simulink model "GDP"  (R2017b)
settings: Solver=FixedStepDiscrete  StartTime=0.0  StopTime=10.0  FixedStep=0.01  RelTol=1e-3  EnableMultiTasking=on
undefined symbols (not defined in the file): ASWTYPE_FALSE, ASWTYPE_TRUE, CcGDP_DCCANBusOffFltTi_ms, Enum_DCCDCConnSt, Enum_LDPCC2St, GDP_CONST1_NUMB, GDP_RUNTIME_MS
libraries: AIWAYS_Powertrain_BMS_lib x68
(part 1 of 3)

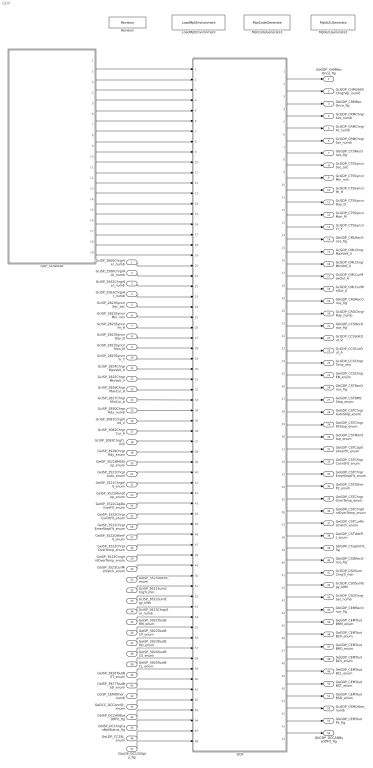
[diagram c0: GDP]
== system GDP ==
  GcISP_2600ChrgrVer_numb : Inport
  GcISP_2560ChrgrAck_numb : Inport  Port=2
  GcISP_2561ChrgrSer_numb : Inport  Port=3
  GcISP_2562ChrgrAr_numb : Inport  Port=4
  GcISP_2823SyncnSec_sec : Inport  Port=5
  GcISP_2823SyncnMin_min : Inport  Port=6
  GcISP_2823SyncnHr_H : Inport  Port=7
  GcISP_2823SyncnDay_D : Inport  Port=8
  GcISP_2823SyncnMon_M : Inport  Port=9
  GcISP_2823SyncnYr_Y : Inport  Port=10
  GcISP_2824ChrgrMaxVolt_V : Inport  Port=11
  GcISP_2825ChrgrMinVolt_V : Inport  Port=12
  GcISP_2826ChrgrMaxCur_A : Inport  Port=13
  GcISP_2827ChrgrMinCur_A : Inport  Port=14
  GcISP_2830ChrgrRdy_numb : Inport  Port=15
  GcISP_3081ChrgrVolt_V : Inport  Port=16
  GcISP_3082ChrgrCur_A : Inport  Port=17
  GcISP_3083ChrgTi_min : Inport  Port=18
  GeISP_3929ChrgrRdy_enum : Inport  Port=19
  GeISP_3521BMSStop_enum : Inport  Port=20
  GeISP_3521ChrgrAuto_enum : Inport  Port=21
  GeISP_3521ChrgrFlt_enum : Inport  Port=22
  GeISP_3521ManStop_enum : Inport  Port=23
  GeISP_3522CapDeliverFlt_enum : Inport  Port=24
  GeISP_3522ChrgrConntFlt_enum : Inport  Port=25
  GeISP_3522ChrgrEmerStopFlt_enum : Inport  Port=26
  GeISP_3522OtherFlt_enum : Inport  Port=27
  GeISP_3522ChrgrOverTemp_enum : Inport  Port=28
  GeISP_3522ChrgrIntOverTemp_enum : Inport  Port=29
  GeISP_3523CurMismatch_enum : Inport  Port=30
  GeISP_3523VoltFlt_enum : Inport  Port=31
  GcISP_3611SumChrgTi_min : Inport  Port=32
  GcISP_3612SumEgy_kWh : Inport  Port=33
  GcISP_3613ChrgrSer_numb : Inport  Port=34
  GeISP_3921ToutBRM_enum : Inport  Port=35
  GeISP_3922ToutBCP_enum : Inport  Port=36
  GeISP_3923ToutBRO_enum : Inport  Port=37
  GeISP_3924ToutBCS_enum : Inport  Port=38
  GeISP_3925ToutBCL_enum : Inport  Port=39
  GeISP_3926ToutBST_enum : Inport  Port=40
  GeISP_3927ToutBSD_enum : Inport  Port=41
  GcISP_CEMOther_numb : Inport  Port=42
  GeDCC_DCConnSt_enum : Inport  Port=43
  GbISP_DCCANBusOffFlt_flg : Inport  Port=44
  GbISP_DCChrgCanNetStatus_flg : Inport  Port=45
  GeLDP_CC2St_enum : Inport  Port=46
  GbLDP_DC12VSply_flg : Inport  Port=47
  DCR : Subsystem
  GDP_Schedule : Stateflow chart  TreatAsAtomicUnit=on
  LoadMptEnvironment : AIWAYS_Powertrain_BMS_lib/Config/LoadMptEnvironment  ProjectName=Comm  SuppierID=NewPlatformUAES
  MptA2LGenerate1 : AIWAYS_Powertrain_BMS_lib/Config/MptA2LGenerate  SystemSampleTime=-1
  MptCodeGenerate1 : AIWAYS_Powertrain_BMS_lib/Config/MptCodeGenerate  SystemSampleTime=-1
  Revision : AIWAYS_Powertrain_BMS_lib/Config/Revision  curVersion='M100C100'  newVersion='M100C100'
  GbGDP_CHMRecOnce_flg : Outport
  GcGDP_CHM2600ChrgrVer_numb : Outport  Port=2
  GbGDP_CRMRecOnce_flg : Outport  Port=3
  GcGDP_CRMChrgrAck_numb : Outport  Port=4
  GcGDP_CRMChrgrAr_numb : Outport  Port=5
  GcGDP_CRMChrgrSer_numb : Outport  Port=6
  GbGDP_CTSRecOnce_flg : Outport  Port=7
  GcGDP_CTSSyncnSec_sec : Outport  Port=8
  GcGDP_CTSSyncnMin_min : Outport  Port=9
  GcGDP_CTSSyncnHr_H : Outport  Port=10
  GcGDP_CTSSyncnDay_D : Outport  Port=11
  GcGDP_CTSSyncnMon_M : Outport  Port=12
  GcGDP_CTSSyncnYr_Y : Outport  Port=13
  GbGDP_CMLRecOnce_flg : Outport  Port=14
  GcGDP_CMLChrgrMaxVolt_V : Outport  Port=15
  GcGDP_CMLChrgrMinVolt_V : Outport  Port=16
  GcGDP_CMLCurMaxOut_A : Outport  Port=17
  GcGDP_CMLCurMinOut_A : Outport  Port=18
  GbGDP_CRORecOnce_flg : Outport  Port=19
  GcGDP_CROChrgrRdy_numb : Outport  Port=20
  GbGDP_CCSRecOnce_flg : Outport  Port=21
  GcGDP_CCSVoltOut_V : Outport  Port=22
  GcGDP_CCSCurOut_A : Outport  Port=23
  GcGDP_CCSChrgrTime_min : Outport  Port=24
  GeGDP_CCSChrgrEN_enum : Outport  Port=25
  GbGDP_CSTRecOnce_flg : Outport  Port=26
  GeGDP_CSTBMSStop_enum : Outport  Port=27
  GeGDP_CSTChrgrAutoStop_enum : Outport  Port=28
  GeGDP_CSTChrgrFltStop_enum : Outport  Port=29
  GeGDP_CSTManStop_enum : Outport  Port=30
  GeGDP_CSTCapDeliverFlt_enum : Outport  Port=31
  GeGDP_CSTChrgrConntFlt_enum : Outport  Port=32
  GeGDP_CSTChrgrEmerStopFlt_enum : Outport  Port=33
  GeGDP_CSTOtherFlt_enum : Outport  Port=34
  GeGDP_CSTChrgrOverTemp_enum : Outport  Port=35
  GeGDP_CSTChrgrIntOverTemp_enum : Outport  Port=36
  GeGDP_CSTCurMismatch_enum : Outport  Port=37
  GeGDP_CSTVoltFlt_enum : Outport  Port=38
  GbGDP_ChrgrInFlt_flg : Outport  Port=39
  GbGDP_CSDRecOnce_flg : Outport  Port=40
  GcGDP_CSDSumChrgTi_min : Outport  Port=41
  GcGDP_CSDSumEgy_kWh : Outport  Port=42
  GcGDP_CSDChrgrSer_numb : Outport  Port=43
  GbGDP_CEMRecOnce_flg : Outport  Port=44
  GeGDP_CEMToutBRM_enum : Outport  Port=45
  GeGDP_CEMToutBCP_enum : Outport  Port=46
  GeGDP_CEMToutBRO_enum : Outport  Port=47
  GeGDP_CEMToutBCS_enum : Outport  Port=48
  GeGDP_CEMToutBCL_enum : Outport  Port=49
  GeGDP_CEMToutBST_enum : Outport  Port=50
  GeGDP_CEMToutBSD_enum : Outport  Port=51
  GcGDP_CEMOther_numb : Outport  Port=52
  GbGDP_CEMToutFlt_flg : Outport  Port=53
  GbGDP_DCCANBusOffFlt_flg : Outport  Port=54
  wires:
  GeISP_3926ToutBST_enum/1 -> DCR/59(GeISP_3926ToutBST_enum)
  GeISP_3921ToutBRM_enum/1 -> DCR/54(GeISP_3921ToutBRM_enum)
  GcISP_2824ChrgrMaxVolt_V/1 -> DCR/30(GcISP_2824ChrgrMaxVolt_V)
  GeISP_3929ChrgrRdy_enum/1 -> DCR/38(GeISP_3929ChrgrRdy_enum)
  GcISP_2827ChrgrMinCur_A/1 -> DCR/33(GcISP_2827ChrgrMinCur_A)
  GcISP_2830ChrgrRdy_numb/1 -> DCR/34(GcISP_2830ChrgrRdy_numb)
  GeISP_3522ChrgrConntFlt_enum/1 -> DCR/44(GeISP_3522ChrgrConntFlt_enum)
  GcISP_3611SumChrgTi_min/1 -> DCR/51(GcISP_3611SumChrgTi_min)
  GcISP_2823SyncnYr_Y/1 -> DCR/29(GcISP_2823SyncnYr_Y)
  GeISP_3521ManStop_enum/1 -> DCR/42(GeISP_3521ManStop_enum)
  GeISP_3522ChrgrIntOverTemp_enum/1 -> DCR/48(GeISP_3522ChrgrIntOverTemp_enum)
  GcISP_3081ChrgrVolt_V/1 -> DCR/35(GcISP_3081ChrgrVolt_V)
  GcISP_2823SyncnHr_H/1 -> DCR/26(GcISP_2823SyncnHr_H)
  GcISP_3613ChrgrSer_numb/1 -> DCR/53(GcISP_3613ChrgrSer_numb)
  GeISP_3522CapDeliverFlt_enum/1 -> DCR/43(GeISP_3522CapDeliverFlt_enum)
  GeISP_3523CurMismatch_enum/1 -> DCR/49(GeISP_3523CurMismatch_enum)
  GeISP_3521BMSStop_enum/1 -> DCR/39(GeISP_3521BMSStop_enum)
  GeISP_3521ChrgrAuto_enum/1 -> DCR/40(GeISP_3521ChrgrAuto_enum)
  GeISP_3925ToutBCL_enum/1 -> DCR/58(GeISP_3925ToutBCL_enum)
  GcISP_2561ChrgrSer_numb/1 -> DCR/22(GcISP_2561ChrgrSer_numb)
  GcISP_2823SyncnMin_min/1 -> DCR/25(GcISP_2823SyncnMin_min)
  GcISP_2823SyncnDay_D/1 -> DCR/27(GcISP_2823SyncnDay_D)
  GcISP_2600ChrgrVer_numb/1 -> DCR/20(GcISP_2600ChrgrVer_numb)
  GcISP_2825ChrgrMinVolt_V/1 -> DCR/31(GcISP_2825ChrgrMinVolt_V)
  GeISP_3923ToutBRO_enum/1 -> DCR/56(GeISP_3923ToutBRO_enum)
  GcISP_2562ChrgrAr_numb/1 -> DCR/23(GcISP_2562ChrgrAr_numb)
  GcISP_2823SyncnSec_sec/1 -> DCR/24(GcISP_2823SyncnSec_sec)
  GcISP_2823SyncnMon_M/1 -> DCR/28(GcISP_2823SyncnMon_M)
  GeISP_3522OtherFlt_enum/1 -> DCR/46(GeISP_3522OtherFlt_enum)
  GcISP_2826ChrgrMaxCur_A/1 -> DCR/32(GcISP_2826ChrgrMaxCur_A)
  GeISP_3521ChrgrFlt_enum/1 -> DCR/41(GeISP_3521ChrgrFlt_enum)
  GeISP_3522ChrgrOverTemp_enum/1 -> DCR/47(GeISP_3522ChrgrOverTemp_enum)
  GeISP_3522ChrgrEmerStopFlt_enum/1 -> DCR/45(GeISP_3522ChrgrEmerStopFlt_enum)
  GcISP_2560ChrgrAck_numb/1 -> DCR/21(GcISP_2560ChrgrAck_numb)
  GcISP_3083ChrgTi_min/1 -> DCR/37(GcISP_3083ChrgTi_min)
  GeISP_3523VoltFlt_enum/1 -> DCR/50(GeISP_3523VoltFlt_enum)
  GcISP_3612SumEgy_kWh/1 -> DCR/52(GcISP_3612SumEgy_kWh)
  GcISP_3082ChrgrCur_A/1 -> DCR/36(GcISP_3082ChrgrCur_A)
  GeISP_3922ToutBCP_enum/1 -> DCR/55(GeISP_3922ToutBCP_enum)
  GeISP_3924ToutBCS_enum/1 -> DCR/57(GeISP_3924ToutBCS_enum)
  GeISP_3927ToutBSD_enum/1 -> DCR/60(GeISP_3927ToutBSD_enum)
  GeDCC_DCConnSt_enum/1 -> DCR/62(GeDCC_DCConnSt_enum)
  GbISP_DCCANBusOffFlt_flg/1 -> DCR/63(GbISP_DCCANBusOffFlt_flg)
  GcISP_CEMOther_numb/1 -> DCR/61(GcISP_CEMOther_numb)
  DCR/14(GbGDP_CMLRecOnce_flg) -> GbGDP_CMLRecOnce_flg/1
  DCR/15(GcGDP_CMLChrgrMaxVolt_V) -> GcGDP_CMLChrgrMaxVolt_V/1
  DCR/16(GcGDP_CMLChrgrMinVolt_V) -> GcGDP_CMLChrgrMinVolt_V/1
  DCR/17(GcGDP_CMLCurMaxOut_A) -> GcGDP_CMLCurMaxOut_A/1
  DCR/18(GcGDP_CMLCurMinOut_A) -> GcGDP_CMLCurMinOut_A/1
  DCR/19(GbGDP_CRORecOnce_flg) -> GbGDP_CRORecOnce_flg/1
  DCR/20(GcGDP_CROChrgrRdy_numb) -> GcGDP_CROChrgrRdy_numb/1
  DCR/21(GbGDP_CCSRecOnce_flg) -> GbGDP_CCSRecOnce_flg/1
  DCR/22(GcGDP_CCSVoltOut_V) -> GcGDP_CCSVoltOut_V/1
  DCR/23(GcGDP_CCSCurOut_A) -> GcGDP_CCSCurOut_A/1
  DCR/24(GcGDP_CCSChrgrTime_min) -> GcGDP_CCSChrgrTime_min/1
  DCR/25(GeGDP_CCSChrgrEN_enum) -> GeGDP_CCSChrgrEN_enum/1
  DCR/26(GbGDP_CSTRecOnce_flg) -> GbGDP_CSTRecOnce_flg/1
  DCR/27(GeGDP_CSTBMSStop_enum) -> GeGDP_CSTBMSStop_enum/1
  DCR/28(GeGDP_CSTChrgrAutoStop_enum) -> GeGDP_CSTChrgrAutoStop_enum/1
  DCR/29(GeGDP_CSTChrgrFltStop_enum) -> GeGDP_CSTChrgrFltStop_enum/1
  DCR/30(GeGDP_CSTManStop_enum) -> GeGDP_CSTManStop_enum/1
  DCR/31(GeGDP_CSTCapDeliverFlt_enum) -> GeGDP_CSTCapDeliverFlt_enum/1
  DCR/32(GeGDP_CSTChrgrConntFlt_enum) -> GeGDP_CSTChrgrConntFlt_enum/1
  DCR/33(GeGDP_CSTChrgrEmerStopFlt_enum) -> GeGDP_CSTChrgrEmerStopFlt_enum/1
  DCR/34(GeGDP_CSTOtherFlt_enum) -> GeGDP_CSTOtherFlt_enum/1
  DCR/35(GeGDP_CSTChrgrOverTemp_enum) -> GeGDP_CSTChrgrOverTemp_enum/1
  DCR/36(GeGDP_CSTChrgrIntOverTemp_enum) -> GeGDP_CSTChrgrIntOverTemp_enum/1
  DCR/37(GeGDP_CSTCurMismatch_enum) -> GeGDP_CSTCurMismatch_enum/1
  DCR/38(GeGDP_CSTVoltFlt_enum) -> GeGDP_CSTVoltFlt_enum/1
  DCR/39(GbGDP_ChrgrInFlt_flg) -> GbGDP_ChrgrInFlt_flg/1
  DCR/40(GbGDP_CSDRecOnce_flg) -> GbGDP_CSDRecOnce_flg/1
  DCR/41(GcGDP_CSDSumChrgTi_min) -> GcGDP_CSDSumChrgTi_min/1
  DCR/42(GcGDP_CSDSumEgy_kWh) -> GcGDP_CSDSumEgy_kWh/1
  DCR/43(GcGDP_CSDChrgrSer_numb) -> GcGDP_CSDChrgrSer_numb/1
  DCR/44(GbGDP_CEMRecOnce_flg) -> GbGDP_CEMRecOnce_flg/1
  DCR/45(GeGDP_CEMToutBRM_enum) -> GeGDP_CEMToutBRM_enum/1
  DCR/46(GeGDP_CEMToutBCP_enum) -> GeGDP_CEMToutBCP_enum/1
  DCR/47(GeGDP_CEMToutBRO_enum) -> GeGDP_CEMToutBRO_enum/1
  DCR/48(GeGDP_CEMToutBCS_enum) -> GeGDP_CEMToutBCS_enum/1
  DCR/49(GeGDP_CEMToutBCL_enum) -> GeGDP_CEMToutBCL_enum/1
  DCR/50(GeGDP_CEMToutBST_enum) -> GeGDP_CEMToutBST_enum/1
  DCR/51(GeGDP_CEMToutBSD_enum) -> GeGDP_CEMToutBSD_enum/1
  DCR/52(GcGDP_CEMOther_numb) -> GcGDP_CEMOther_numb/1
  DCR/53(GbGDP_CEMToutFlt_flg) -> GbGDP_CEMToutFlt_flg/1
  DCR/54(GbGDP_DCCANBusOffFlt_flg) -> GbGDP_DCCANBusOffFlt_flg/1
  DCR/1(GbGDP_CHMRecOnce_flg) -> GbGDP_CHMRecOnce_flg/1
  DCR/2(GcGDP_CHM2600ChrgrVer_numb) -> GcGDP_CHM2600ChrgrVer_numb/1
  DCR/3(GbGDP_CRMRecOnce_flg) -> GbGDP_CRMRecOnce_flg/1
  DCR/4(GcGDP_CRMChrgrAck_numb) -> GcGDP_CRMChrgrAck_numb/1
  DCR/5(GcGDP_CRMChrgrAr_numb) -> GcGDP_CRMChrgrAr_numb/1
  DCR/6(GcGDP_CRMChrgrSer_numb) -> GcGDP_CRMChrgrSer_numb/1
  DCR/7(GbGDP_CTSRecOnce_flg) -> GbGDP_CTSRecOnce_flg/1
  DCR/8(GcGDP_CTSSyncnSec_sec) -> GcGDP_CTSSyncnSec_sec/1
  DCR/9(GcGDP_CTSSyncnMin_min) -> GcGDP_CTSSyncnMin_min/1
  DCR/10(GcGDP_CTSSyncnHr_H) -> GcGDP_CTSSyncnHr_H/1
  DCR/11(GcGDP_CTSSyncnDay_D) -> GcGDP_CTSSyncnDay_D/1
  DCR/12(GcGDP_CTSSyncnMon_M) -> GcGDP_CTSSyncnMon_M/1
  DCR/13(GcGDP_CTSSyncnYr_Y) -> GcGDP_CTSSyncnYr_Y/1
  GbISP_DCChrgCanNetStatus_flg/1 -> DCR/64(GbISP_DCChrgCanNetStatus_flg)
  GeLDP_CC2St_enum/1 -> DCR/65(GeLDP_CC2St_enum)
  GbLDP_DC12VSply_flg/1 -> DCR/66(GbLDP_DC12VSply_flg)
  GDP_Schedule/1(GDP_CHM_250ms()) -> DCR/1(GDP_CHM_250ms)
  GDP_Schedule/2(GDP_CRM_250ms()) -> DCR/2(GDP_CRM_250ms)
  GDP_Schedule/3(GDP_CTS_500ms()) -> DCR/3(GDP_CTS_500ms)
  GDP_Schedule/4(GDP_CML_500ms()) -> DCR/4(GDP_CML_500ms)
  GDP_Schedule/5(GDP_CRO_50ms()) -> DCR/5(GDP_CRO_50ms)
  GDP_Schedule/6(GDP_CCS_50ms()) -> DCR/6(GDP_CCS_50ms)
  GDP_Schedule/8(GDP_CSD_250ms()) -> DCR/8(GDP_CSD_250ms)
  GDP_Schedule/9(GDP_CEM_250ms()) -> DCR/9(GDP_CEM_250ms)
  GDP_Schedule/10(GDP_BusOff_10ms()) -> DCR/10(GDP_BusOff_10ms)
  GDP_Schedule/11(GDP_CCSUpdateClr_50ms()) -> DCR/11(GDP_CCSUpdateClr_50ms)
  GDP_Schedule/12(GDP_CEMUpdateClr_250ms()) -> DCR/12(GDP_CEMUpdateClr_250ms)
  GDP_Schedule/13(GDP_CHMUpdateClr_250ms()) -> DCR/13(GDP_CHMUpdateClr_250ms)
  GDP_Schedule/14(GDP_CMLUpdateClr_500ms()) -> DCR/14(GDP_CMLUpdateClr_500ms)
  GDP_Schedule/16(GDP_CROUpdateClr_50ms()) -> DCR/16(GDP_CROUpdateClr_50ms)
  GDP_Schedule/15(GDP_CRMUpdateClr_250ms()) -> DCR/15(GDP_CRMUpdateClr_250ms)
  GDP_Schedule/17(GDP_CSDUpdateClr_250ms()) -> DCR/17(GDP_CSDUpdateClr_250ms)
  GDP_Schedule/18(GDP_CSTUpdateClr_10ms()) -> DCR/18(GDP_CSTUpdateClr_10ms)
  GDP_Schedule/19(GDP_CTSUpdateClr_500ms()) -> DCR/19(GDP_CTSUpdateClr_500ms)
  GDP_Schedule/7(GDP_CST_10ms()) -> DCR/7(GDP_CST_10ms)

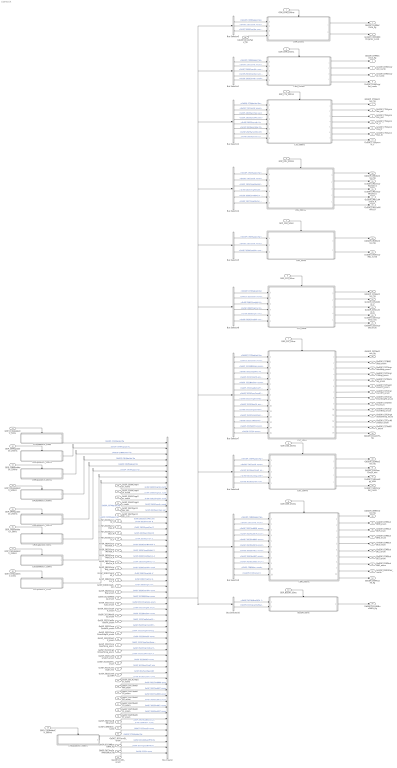
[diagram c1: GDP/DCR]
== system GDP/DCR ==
  GDP_CHM_250ms : Inport
  GDP_CRM_250ms : Inport  Port=2
  GDP_CTS_500ms : Inport  Port=3
  GDP_CML_500ms : Inport  Port=4
  GDP_CRO_50ms : Inport  Port=5
  GDP_CCS_50ms : Inport  Port=6
  GDP_CST_10ms : Inport  Port=7
  GDP_CSD_250ms : Inport  Port=8
  GDP_CEM_250ms : Inport  Port=9
  GDP_BusOff_10ms : Inport  Port=10
  GDP_CCSUpdateClr_50ms : Inport  Port=11
  GDP_CEMUpdateClr_250ms : Inport  Port=12
  GDP_CHMUpdateClr_250ms : Inport  Port=13
  GDP_CMLUpdateClr_500ms : Inport  Port=14
  GDP_CRMUpdateClr_250ms : Inport  Port=15
  GDP_CROUpdateClr_50ms : Inport  Port=16
  GDP_CSDUpdateClr_250ms : Inport  Port=17
  GDP_CSTUpdateClr_10ms : Inport  Port=18
  GDP_CTSUpdateClr_500ms : Inport  Port=19
  GcISP_2600ChrgrVer_numb : Inport  Port=20
  GcISP_2560ChrgrAck_numb : Inport  Port=21
  GcISP_2561ChrgrSer_numb : Inport  Port=22
  GcISP_2562ChrgrAr_numb : Inport  Port=23
  GcISP_2823SyncnSec_sec : Inport  Port=24
  GcISP_2823SyncnMin_min : Inport  Port=25
  GcISP_2823SyncnHr_H : Inport  Port=26
  GcISP_2823SyncnDay_D : Inport  Port=27
  GcISP_2823SyncnMon_M : Inport  Port=28
  GcISP_2823SyncnYr_Y : Inport  Port=29
  GcISP_2824ChrgrMaxVolt_V : Inport  Port=30
  GcISP_2825ChrgrMinVolt_V : Inport  Port=31
  GcISP_2826ChrgrMaxCur_A : Inport  Port=32
  GcISP_2827ChrgrMinCur_A : Inport  Port=33
  GcISP_2830ChrgrRdy_numb : Inport  Port=34
  GcISP_3081ChrgrVolt_V : Inport  Port=35
  GcISP_3082ChrgrCur_A : Inport  Port=36
  GcISP_3083ChrgTi_min : Inport  Port=37
  GeISP_3929ChrgrRdy_enum : Inport  Port=38
  GeISP_3521BMSStop_enum : Inport  Port=39
  GeISP_3521ChrgrAuto_enum : Inport  Port=40
  GeISP_3521ChrgrFlt_enum : Inport  Port=41
  GeISP_3521ManStop_enum : Inport  Port=42
  GeISP_3522CapDeliverFlt_enum : Inport  Port=43
  GeISP_3522ChrgrConntFlt_enum : Inport  Port=44
  GeISP_3522ChrgrEmerStopFlt_enum : Inport  Port=45
  GeISP_3522OtherFlt_enum : Inport  Port=46
  GeISP_3522ChrgrOverTemp_enum : Inport  Port=47
  GeISP_3522ChrgrIntOverTemp_enum : Inport  Port=48
  GeISP_3523CurMismatch_enum : Inport  Port=49
  GeISP_3523VoltFlt_enum : Inport  Port=50
  GcISP_3611SumChrgTi_min : Inport  Port=51
  GcISP_3612SumEgy_kWh : Inport  Port=52
  GcISP_3613ChrgrSer_numb : Inport  Port=53
  GeISP_3921ToutBRM_enum : Inport  Port=54
  GeISP_3922ToutBCP_enum : Inport  Port=55
  GeISP_3923ToutBRO_enum : Inport  Port=56
  GeISP_3924ToutBCS_enum : Inport  Port=57
  GeISP_3925ToutBCL_enum : Inport  Port=58
  GeISP_3926ToutBST_enum : Inport  Port=59
  GeISP_3927ToutBSD_enum : Inport  Port=60
  GcISP_CEMOther_numb : Inport  Port=61
  GeDCC_DCConnSt_enum : Inport  Port=62
  GbISP_DCCANBusOffFlt_flg : Inport  Port=63
  GbISP_DCChrgCanNetStatus_flg : Inport  Port=64
  GeLDP_CC2St_enum : Inport  Port=65
  GbLDP_DC12VSply_flg : Inport  Port=66
  Bus Creator : BusCreator  Inputs=55
  Bus Selector1 : BusSelector  OutputSignals=GbGDP_CRMMsgUpd_flg,GeDCC_DCConnSt_enum,GcISP_2560ChrgrAck_numb,GcISP_2561ChrgrSer_numb,GcISP_2562ChrgrAr_numb
  Bus Selector10 : BusSelector  OutputSignals=GbISP_DCCANBusOffFlt_flg,GbISP_DCChrgCanNetStatus_flg
  Bus Selector2 : BusSelector  OutputSignals=GbGDP_CTSMsgUpd_flg,GeDCC_DCConnSt_enum,GcISP_2823SyncnSec_sec,GcISP_2823SyncnMin_min,GcISP_2823SyncnHr_H,GcISP_2823SyncnDay_D,GcISP_2823SyncnMon_M,GcISP_2823SyncnYr_Y
  Bus Selector3 : BusSelector  OutputSignals=GbGDP_CHMMsgUpd_flg,GeDCC_DCConnSt_enum,GcISP_2600ChrgrVer_numb
  Bus Selector4 : BusSelector  OutputSignals=GbGDP_CMLMsgUpd_flg,GeDCC_DCConnSt_enum,GcISP_2824ChrgrMaxVolt_V,GcISP_2825ChrgrMinVolt_V,GcISP_2826ChrgrMaxCur_A,GcISP_2827ChrgrMinCur_A
  Bus Selector5 : BusSelector  OutputSignals=GbGDP_CROMsgUpd_flg,GeDCC_DCConnSt_enum,GcISP_2830ChrgrRdy_numb
  Bus Selector6 : BusSelector  OutputSignals=GbGDP_CCSMsgUpd_flg,GeDCC_DCConnSt_enum,GcISP_3081ChrgrVolt_V,GcISP_3082ChrgrCur_A,GcISP_3083ChrgTi_min,GeISP_3929ChrgrRdy_enum
  Bus Selector7 : BusSelector  OutputSignals=GbGDP_CSTMsgUpd_flg,GeDCC_DCConnSt_enum,GeISP_3521BMSStop_enum,GeISP_3521ChrgrAuto_enum,GeISP_3521ChrgrFlt_enum,GeISP_3521ManStop_enum,GeISP_3522CapDeliverFlt_enum,GeISP_3522ChrgrConntFlt_enum,GeISP_3522ChrgrEmerStopFlt_enum,GeISP_3522OtherFlt_enum,GeISP_3522ChrgrOverTemp_enum,GeISP_3522ChrgrIntOverTemp_enum,GeISP_3523CurMismatch_enum,GeISP_3523VoltFlt_enum,GeLDP_CC2St_enum
  Bus Selector8 : BusSelector  OutputSignals=GbGDP_CSDMsgUpd_flg,GeDCC_DCConnSt_enum,GcISP_3611SumChrgTi_min,GcISP_3612SumEgy_kWh,GcISP_3613ChrgrSer_numb
  Bus Selector9 : BusSelector  OutputSignals=GbGDP_CEMMsgUpd_flg,GeDCC_DCConnSt_enum,GeISP_3921ToutBRM_enum,GeISP_3922ToutBCP_enum,GeISP_3923ToutBRO_enum,GeISP_3924ToutBCS_enum,GeISP_3925ToutBCL_enum,GeISP_3926ToutBST_enum,GeISP_3927ToutBSD_enum,GcISP_CEMOther_numb,GeLDP_CC2St_enum
  BusOff_10ms : Subsystem
  CCSUpdateClr_50ms : Subsystem
  CCS_50ms : Subsystem
  CEMUpdateClr_250ms : Subsystem
  CEM_250ms : Subsystem
  CHMUpdateClr_250ms : Subsystem
  CHM_250ms : Subsystem
  CMLUpdateClr_500ms : Subsystem
  CML_500ms : Subsystem
  CRMUpdateClr_250ms : Subsystem
  CRM_250ms : Subsystem
  CROUpdateClr_50ms : Subsystem
  CRO_50ms : Subsystem
  CSDUpdateClr_250ms : Subsystem
  CSD_250ms : Subsystem
  CSTUpdateClr_10ms : Subsystem
  CST_10ms : Subsystem
  CTSUpdateClr_500ms : Subsystem
  CTS_500ms : Subsystem
  GbGDP_CHMRecOnce_flg : Outport
  GcGDP_CHM2600ChrgrVer_numb : Outport  Port=2
  GbGDP_CRMRecOnce_flg : Outport  Port=3
  GcGDP_CRMChrgrAck_numb : Outport  Port=4
  GcGDP_CRMChrgrAr_numb : Outport  Port=5
  GcGDP_CRMChrgrSer_numb : Outport  Port=6
  GbGDP_CTSRecOnce_flg : Outport  Port=7
  GcGDP_CTSSyncnSec_sec : Outport  Port=8
  GcGDP_CTSSyncnMin_min : Outport  Port=9
  GcGDP_CTSSyncnHr_H : Outport  Port=10
  GcGDP_CTSSyncnDay_D : Outport  Port=11
  GcGDP_CTSSyncnMon_M : Outport  Port=12
  GcGDP_CTSSyncnYr_Y : Outport  Port=13
  GbGDP_CMLRecOnce_flg : Outport  Port=14
  GcGDP_CMLChrgrMaxVolt_V : Outport  Port=15
  GcGDP_CMLChrgrMinVolt_V : Outport  Port=16
  GcGDP_CMLCurMaxOut_A : Outport  Port=17
  GcGDP_CMLCurMinOut_A : Outport  Port=18
  GbGDP_CRORecOnce_flg : Outport  Port=19
  GcGDP_CROChrgrRdy_numb : Outport  Port=20
  GbGDP_CCSRecOnce_flg : Outport  Port=21
  GcGDP_CCSVoltOut_V : Outport  Port=22
  GcGDP_CCSCurOut_A : Outport  Port=23
  GcGDP_CCSChrgrTime_min : Outport  Port=24
  GeGDP_CCSChrgrEN_enum : Outport  Port=25
  GbGDP_CSTRecOnce_flg : Outport  Port=26
  GeGDP_CSTBMSStop_enum : Outport  Port=27
  GeGDP_CSTChrgrAutoStop_enum : Outport  Port=28
  GeGDP_CSTChrgrFltStop_enum : Outport  Port=29
  GeGDP_CSTManStop_enum : Outport  Port=30
  GeGDP_CSTCapDeliverFlt_enum : Outport  Port=31
  GeGDP_CSTChrgrConntFlt_enum : Outport  Port=32
  GeGDP_CSTChrgrEmerStopFlt_enum : Outport  Port=33
  GeGDP_CSTOtherFlt_enum : Outport  Port=34
  GeGDP_CSTChrgrOverTemp_enum : Outport  Port=35
  GeGDP_CSTChrgrIntOverTemp_enum : Outport  Port=36
  GeGDP_CSTCurMismatch_enum : Outport  Port=37
  GeGDP_CSTVoltFlt_enum : Outport  Port=38
  GbGDP_ChrgrInFlt_flg : Outport  Port=39
  GbGDP_CSDRecOnce_flg : Outport  Port=40
  GcGDP_CSDSumChrgTi_min : Outport  Port=41
  GcGDP_CSDSumEgy_kWh : Outport  Port=42
  GcGDP_CSDChrgrSer_numb : Outport  Port=43
  GbGDP_CEMRecOnce_flg : Outport  Port=44
  GeGDP_CEMToutBRM_enum : Outport  Port=45
  GeGDP_CEMToutBCP_enum : Outport  Port=46
  GeGDP_CEMToutBRO_enum : Outport  Port=47
  GeGDP_CEMToutBCS_enum : Outport  Port=48
  GeGDP_CEMToutBCL_enum : Outport  Port=49
  GeGDP_CEMToutBST_enum : Outport  Port=50
  GeGDP_CEMToutBSD_enum : Outport  Port=51
  GcGDP_CEMOther_numb : Outport  Port=52
  GbGDP_CEMToutFlt_flg : Outport  Port=53
  GbGDP_DCCANBusOffFlt_flg : Outport  Port=54
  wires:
  GcISP_2823SyncnMin_min/1 -> Bus Creator/14  "GcISP_2823SyncnMin_min"
  Bus Selector9/6 -> CEM_250ms/6(GeISP_3924ToutBCS_enum)  "<GeISP_3924ToutBCS_enum>"
  CST_10ms/3(GeGDP_CSTChrgrAutoStop_enum) -> GeGDP_CSTChrgrAutoStop_enum/1
  CEM_250ms/4(GeGDP_CEMToutBRO_enum) -> GeGDP_CEMToutBRO_enum/1
  GeISP_3521ChrgrAuto_enum/1 -> Bus Creator/29  "GeISP_3521ChrgrAuto_enum"
  Bus Selector7/13 -> CST_10ms/13(GeISP_3523CurMismatch_enum)  "<GeISP_3523CurMismatch_enum>"
  Bus Selector9/4 -> CEM_250ms/4(GeISP_3922ToutBCP_enum)  "<GeISP_3922ToutBCP_enum>"
  Bus Selector9/1 -> CEM_250ms/1(GbGDP_CEMMsgUpd_flg)  "<GbGDP_CEMMsgUpd_flg>"
  Bus Selector6/5 -> CCS_50ms/5(GcISP_3083ChrgTi_min)  "<GcISP_3083ChrgTi_min>"
  Bus Selector7/9 -> CST_10ms/9(GeISP_3522ChrgrEmerStopFlt_enum)  "<GeISP_3522ChrgrEmerStopFlt_enum>"
  Bus Selector7/6 -> CST_10ms/6(GeISP_3521ManStop_enum)  "<GeISP_3521ManStop_enum>"
  GDP_CML_500ms/1 -> CML_500ms/Trigger
  CEM_250ms/9(GcGDP_CEMOther_numb) -> GcGDP_CEMOther_numb/1
  Bus Selector1/3 -> CRM_250ms/3(GcISP_2560ChrgrAck_numb)  "<GcISP_2560ChrgrAck_numb>"
  CML_500ms/4(GcGDP_CMLCurMaxOut_A) -> GcGDP_CMLCurMaxOut_A/1
  GeISP_3523VoltFlt_enum/1 -> Bus Creator/39  "GeISP_3523VoltFlt_enum"
  GcISP_3082ChrgrCur_A/1 -> Bus Creator/25  "GcISP_3082ChrgrCur_A"
  Bus Selector9/9 -> CEM_250ms/9(GeISP_3927ToutBSD_enum)  "<GeISP_3927ToutBSD_enum>"
  GcISP_2560ChrgrAck_numb/1 -> Bus Creator/10  "GcISP_2560ChrgrAck_numb"
  CSD_250ms/2(GcGDP_CSDSumChrgTi_min) -> GcGDP_CSDSumChrgTi_min/1
  GeISP_3521BMSStop_enum/1 -> Bus Creator/28  "GeISP_3521BMSStop_enum"
  Bus Selector2/3 -> CTS_500ms/3(GcISP_2823SyncnSec_sec)  "<GcISP_2823SyncnSec_sec>"
  GeISP_3927ToutBSD_enum/1 -> Bus Creator/49  "GeISP_3927ToutBSD_enum"
  GcISP_2827ChrgrMinCur_A/1 -> Bus Creator/22  "GcISP_2827ChrgrMinCur_A"
  CEM_250ms/6(GeGDP_CEMToutBCL_enum) -> GeGDP_CEMToutBCL_enum/1
  CRO_50ms/1(GbGDP_CRORecOnce_flg) -> GbGDP_CRORecOnce_flg/1
  GDP_CEM_250ms/1 -> CEM_250ms/Trigger
  CMLUpdateClr_500ms/1(GbGDP_CMLMsgUpd_flg) -> Bus Creator/4  "GbGDP_CMLMsgUpd_flg"
  Bus Selector3/2 -> CHM_250ms/2(GeDCC_DCConnSt_enum)  "<GeDCC_DCConnSt_enum>"
  CCS_50ms/2(GcGDP_CCSVoltOut_V) -> GcGDP_CCSVoltOut_V/1
  CSD_250ms/4(GcGDP_CSDChrgrSer_numb) -> GcGDP_CSDChrgrSer_numb/1
  Bus Selector4/4 -> CML_500ms/4(GcISP_2825ChrgrMinVolt_V)  "<GcISP_2825ChrgrMinVolt_V>"
  CRMUpdateClr_250ms/1(GbGDP_CRMMsgUpd_flg) -> Bus Creator/5  "GbGDP_CRMMsgUpd_flg"
  Bus Selector7/4 -> CST_10ms/4(GeISP_3521ChrgrAuto_enum)  "<GeISP_3521ChrgrAuto_enum>"
  CST_10ms/12(GeGDP_CSTCurMismatch_enum) -> GeGDP_CSTCurMismatch_enum/1
  Bus Creator/1 -> Bus Selector3/1, Bus Selector1/1, Bus Selector2/1, Bus Selector4/1, Bus Selector5/1, Bus Selector6/1, Bus Selector7/1, Bus Selector8/1, Bus Selector9/1, Bus Selector10/1
  GeISP_3522ChrgrEmerStopFlt_enum/1 -> Bus Creator/34  "GeISP_3522ChrgrEmerStopFlt_enum"
  CML_500ms/5(GcGDP_CMLCurMinOut_A) -> GcGDP_CMLCurMinOut_A/1
  Bus Selector2/1 -> CTS_500ms/1(GbGDP_CTSMsgUpd_flg)  "<GbGDP_CTSMsgUpd_flg>"
  Bus Selector4/3 -> CML_500ms/3(GcISP_2824ChrgrMaxVolt_V)  "<GcISP_2824ChrgrMaxVolt_V>"
  CST_10ms/2(GeGDP_CSTBMSStop_enum) -> GeGDP_CSTBMSStop_enum/1
  CHMUpdateClr_250ms/1(GbGDP_CHMMsgUpd_flg) -> Bus Creator/3  "GbGDP_CHMMsgUpd_flg"
  GcISP_3612SumEgy_kWh/1 -> Bus Creator/41  "GcISP_3612SumEgy_kWh"
  Bus Selector7/5 -> CST_10ms/5(GeISP_3521ChrgrFlt_enum)  "<GeISP_3521ChrgrFlt_enum>"
  CST_10ms/6(GeGDP_CSTCapDeliverFlt_enum) -> GeGDP_CSTCapDeliverFlt_enum/1
  CST_10ms/5(GeGDP_CSTManStop_enum) -> GeGDP_CSTManStop_enum/1
  Bus Selector6/4 -> CCS_50ms/4(GcISP_3082ChrgrCur_A)  "<GcISP_3082ChrgrCur_A>"
  Bus Selector7/7 -> CST_10ms/7(GeISP_3522CapDeliverFlt_enum)  "<GeISP_3522CapDeliverFlt_enum>"
  CEM_250ms/2(GeGDP_CEMToutBRM_enum) -> GeGDP_CEMToutBRM_enum/1
  CML_500ms/1(GbGDP_CMLRecOnce_flg) -> GbGDP_CMLRecOnce_flg/1
  CST_10ms/8(GeGDP_CSTChrgrEmerStopFlt_enum) -> GeGDP_CSTChrgrEmerStopFlt_enum/1
  CST_10ms/9(GeGDP_CSTOtherFlt_enum) -> GeGDP_CSTOtherFlt_enum/1
  Bus Selector6/6 -> CCS_50ms/6(GeISP_3929ChrgrRdy_enum)  "<GeISP_3929ChrgrRdy_enum>"
  GcISP_2823SyncnHr_H/1 -> Bus Creator/15  "GcISP_2823SyncnHr_H"
  GDP_CRO_50ms/1 -> CRO_50ms/Trigger
  GDP_CTS_500ms/1 -> CTS_500ms/Trigger
  GeISP_3522ChrgrIntOverTemp_enum/1 -> Bus Creator/37  "GeISP_3522ChrgrIntOverTemp_enum"
  CRM_250ms/4(GcGDP_CRMChrgrSer_numb) -> GcGDP_CRMChrgrSer_numb/1
  CSD_250ms/3(GcGDP_CSDSumEgy_kWh) -> GcGDP_CSDSumEgy_kWh/1
  CTS_500ms/1(GbGDP_CTSRecOnce_flg) -> GbGDP_CTSRecOnce_flg/1
  CML_500ms/2(GcGDP_CMLChrgrMaxVolt_V) -> GcGDP_CMLChrgrMaxVolt_V/1
  Bus Selector7/12 -> CST_10ms/12(GeISP_3522ChrgrIntOverTemp_enum)  "<GeISP_3522ChrgrIntOverTemp_enum>"
  Bus Selector1/1 -> CRM_250ms/1(GbGDP_CRMMsgUpd_flg)  "<GbGDP_CRMMsgUpd_flg>"
  Bus Selector7/14 -> CST_10ms/14(GeISP_3523VoltFlt_enum)  "<GeISP_3523VoltFlt_enum>"
  CTS_500ms/6(GcGDP_CTSSyncnMon_M) -> GcGDP_CTSSyncnMon_M/1
  Bus Selector7/1 -> CST_10ms/1(GbGDP_CSTMsgUpd_flg)  "<GbGDP_CSTMsgUpd_flg>"
  GcISP_2826ChrgrMaxCur_A/1 -> Bus Creator/21  "GcISP_2826ChrgrMaxCur_A"
  GcISP_2825ChrgrMinVolt_V/1 -> Bus Creator/20  "GcISP_2825ChrgrMinVolt_V"
  CST_10ms/7(GeGDP_CSTChrgrConntFlt_enum) -> GeGDP_CSTChrgrConntFlt_enum/1
  GeISP_3522OtherFlt_enum/1 -> Bus Creator/35  "GeISP_3522OtherFlt_enum"
  GeISP_3922ToutBCP_enum/1 -> Bus Creator/44  "GeISP_3922ToutBCP_enum"
  GeISP_3929ChrgrRdy_enum/1 -> Bus Creator/27  "GeISP_3929ChrgrRdy_enum"
  CST_10ms/4(GeGDP_CSTChrgrFltStop_enum) -> GeGDP_CSTChrgrFltStop_enum/1
  GcISP_3613ChrgrSer_numb/1 -> Bus Creator/42  "GcISP_3613ChrgrSer_numb"
  GDP_CRM_250ms/1 -> CRM_250ms/Trigger
  GeISP_3926ToutBST_enum/1 -> Bus Creator/48  "GeISP_3926ToutBST_enum"
  CST_10ms/13(GeGDP_CSTVoltFlt_enum) -> GeGDP_CSTVoltFlt_enum/1
  Bus Selector8/2 -> CSD_250ms/2(GeDCC_DCConnSt_enum)  "<GeDCC_DCConnSt_enum>"
  Bus Selector6/1 -> CCS_50ms/1(GbGDP_CCSMsgUpd_flg)  "<GbGDP_CCSMsgUpd_flg>"
  CEM_250ms/5(GeGDP_CEMToutBCS_enum) -> GeGDP_CEMToutBCS_enum/1
  Bus Selector9/2 -> CEM_250ms/2(GeDCC_DCConnSt_enum)  "<GeDCC_DCConnSt_enum>"
  CCS_50ms/5(GeGDP_CCSChrgrEN_enum) -> GeGDP_CCSChrgrEN_enum/1
  CEM_250ms/7(GeGDP_CEMToutBST_enum) -> GeGDP_CEMToutBST_enum/1
  Bus Selector8/1 -> CSD_250ms/1(GbGDP_CSDMsgUpd_flg)  "<GbGDP_CSDMsgUpd_flg>"
  GcISP_2600ChrgrVer_numb/1 -> Bus Creator/9  "GcISP_2600ChrgrVer_numb"
  Bus Selector6/2 -> CCS_50ms/2(GeDCC_DCConnSt_enum)  "<GeDCC_DCConnSt_enum>"
  GcISP_2823SyncnYr_Y/1 -> Bus Creator/18  "GcISP_2823SyncnYr_Y"
  CTS_500ms/5(GcGDP_CTSSyncnDay_D) -> GcGDP_CTSSyncnDay_D/1
  GDP_CEMUpdateClr_250ms/1 -> CEMUpdateClr_250ms/Trigger
  GeISP_3522ChrgrOverTemp_enum/1 -> Bus Creator/36  "GeISP_3522ChrgrOverTemp_enum"
  Bus Selector7/11 -> CST_10ms/11(GeISP_3522ChrgrOverTemp_enum)  "<GeISP_3522ChrgrOverTemp_enum>"
  Bus Selector1/4 -> CRM_250ms/4(GcISP_2561ChrgrSer_numb)  "<GcISP_2561ChrgrSer_numb>"
  Bus Selector8/4 -> CSD_250ms/4(GcISP_3612SumEgy_kWh)  "<GcISP_3612SumEgy_kWh>"
  CSD_250ms/1(GbGDP_CSDRecOnce_flg) -> GbGDP_CSDRecOnce_flg/1
  CSTUpdateClr_10ms/1(GbGDP_CSTMsgUpd_flg) -> Bus Creator/8  "GbGDP_CSTMsgUpd_flg"
  CEM_250ms/1(GbGDP_CEMRecOnce_flg) -> GbGDP_CEMRecOnce_flg/1
  Bus Selector4/2 -> CML_500ms/2(GeDCC_DCConnSt_enum)  "<GeDCC_DCConnSt_enum>"
  CST_10ms/11(GeGDP_CSTChrgrIntOverTemp_enum) -> GeGDP_CSTChrgrIntOverTemp_enum/1
  GcISP_3083ChrgTi_min/1 -> Bus Creator/26  "GcISP_3083ChrgTi_min"
  GcISP_CEMOther_numb/1 -> Bus Creator/50  "GcISP_CEMOther_numb"
  GbISP_DCCANBusOffFlt_flg/1 -> Bus Creator/53  "GbISP_DCCANBusOffFlt_flg"
  Bus Selector7/2 -> CST_10ms/2(GeDCC_DCConnSt_enum)  "<GeDCC_DCConnSt_enum>"
  Bus Selector4/5 -> CML_500ms/5(GcISP_2826ChrgrMaxCur_A)  "<GcISP_2826ChrgrMaxCur_A>"
  Bus Selector4/6 -> CML_500ms/6(GcISP_2827ChrgrMinCur_A)  "<GcISP_2827ChrgrMinCur_A>"
  Bus Selector3/3 -> CHM_250ms/3(GcISP_2600ChrgrVer_numb)  "<GcISP_2600ChrgrVer_numb>"
  CEMUpdateClr_250ms/1(GbGDP_CEMMsgUpd_flg) -> Bus Creator/2  "GbGDP_CEMMsgUpd_flg"
  Bus Selector1/2 -> CRM_250ms/2(GeDCC_DCConnSt_enum)  "<GeDCC_DCConnSt_enum>"
  GcISP_2823SyncnSec_sec/1 -> Bus Creator/13  "GcISP_2823SyncnSec_sec"
  Bus Selector4/1 -> CML_500ms/1(GbGDP_CMLMsgUpd_flg)  "<GbGDP_CMLMsgUpd_flg>"
  CHM_250ms/1(GbGDP_CHMRecOnce_flg) -> GbGDP_CHMRecOnce_flg/1
  Bus Selector1/5 -> CRM_250ms/5(GcISP_2562ChrgrAr_numb)  "<GcISP_2562ChrgrAr_numb>"
  Bus Selector6/3 -> CCS_50ms/3(GcISP_3081ChrgrVolt_V)  "<GcISP_3081ChrgrVolt_V>"
  Bus Selector9/7 -> CEM_250ms/7(GeISP_3925ToutBCL_enum)  "<GeISP_3925ToutBCL_enum>"
  GDP_CMLUpdateClr_500ms/1 -> CMLUpdateClr_500ms/Trigger
  CST_10ms/1(GbGDP_CSTRecOnce_flg) -> GbGDP_CSTRecOnce_flg/1
  BusOff_10ms/1(GbGDP_DCCANBusOffFlt_flg) -> GbGDP_DCCANBusOffFlt_flg/1
  GeISP_3925ToutBCL_enum/1 -> Bus Creator/47  "GeISP_3925ToutBCL_enum"
  Bus Selector5/2 -> CRO_50ms/2(GeDCC_DCConnSt_enum)  "<GeDCC_DCConnSt_enum>"
  GcISP_3611SumChrgTi_min/1 -> Bus Creator/40  "GcISP_3611SumChrgTi_min"
  Bus Selector7/8 -> CST_10ms/8(GeISP_3522ChrgrConntFlt_enum)  "<GeISP_3522ChrgrConntFlt_enum>"
  CHM_250ms/2(GcGDP_CHM2600ChrgrVer_numb) -> GcGDP_CHM2600ChrgrVer_numb/1
  GeISP_3923ToutBRO_enum/1 -> Bus Creator/45  "GeISP_3923ToutBRO_enum"
  GcISP_3081ChrgrVolt_V/1 -> Bus Creator/24  "GcISP_3081ChrgrVolt_V"
  CCS_50ms/1(GbGDP_CCSRecOnce_flg) -> GbGDP_CCSRecOnce_flg/1
  CTS_500ms/2(GcGDP_CTSSyncnSec_sec) -> GcGDP_CTSSyncnSec_sec/1
  CRM_250ms/3(GcGDP_CRMChrgrAr_numb) -> GcGDP_CRMChrgrAr_numb/1
  CSDUpdateClr_250ms/1(GbGDP_CSDMsgUpd_flg) -> Bus Creator/7  "GbGDP_CSDMsgUpd_flg"
  Bus Selector2/8 -> CTS_500ms/8(GcISP_2823SyncnYr_Y)  "<GcISP_2823SyncnYr_Y>"
  GDP_CSD_250ms/1 -> CSD_250ms/Trigger
  CRM_250ms/1(GbGDP_CRMRecOnce_flg) -> GbGDP_CRMRecOnce_flg/1
  Bus Selector9/5 -> CEM_250ms/5(GeISP_3923ToutBRO_enum)  "<GeISP_3923ToutBRO_enum>"
  GcISP_2830ChrgrRdy_numb/1 -> Bus Creator/23  "GcISP_2830ChrgrRdy_numb"
  CCS_50ms/4(GcGDP_CCSChrgrTime_min) -> GcGDP_CCSChrgrTime_min/1
  CRM_250ms/2(GcGDP_CRMChrgrAck_numb) -> GcGDP_CRMChrgrAck_numb/1
  Bus Selector5/1 -> CRO_50ms/1(GbGDP_CROMsgUpd_flg)  "<GbGDP_CROMsgUpd_flg>"
  GeISP_3521ManStop_enum/1 -> Bus Creator/31  "GeISP_3521ManStop_enum"
  Bus Selector2/6 -> CTS_500ms/6(GcISP_2823SyncnDay_D)  "<GcISP_2823SyncnDay_D>"
  GeDCC_DCConnSt_enum/1 -> Bus Creator/51  "GeDCC_DCConnSt_enum"
  Bus Selector9/10 -> CEM_250ms/10(GcISP_CEMOther_numb)  "<GcISP_CEMOther_numb>"
  CML_500ms/3(GcGDP_CMLChrgrMinVolt_V) -> GcGDP_CMLChrgrMinVolt_V/1
  Bus Selector10/1 -> BusOff_10ms/1(GbISP_DCCANBusOffFlt_flg)  "<GbISP_DCCANBusOffFlt_flg>"
  CRO_50ms/2(GcGDP_CROChrgrRdy_numb) -> GcGDP_CROChrgrRdy_numb/1
  Bus Selector7/3 -> CST_10ms/3(GeISP_3521BMSStop_enum)  "<GeISP_3521BMSStop_enum>"
  CCSUpdateClr_50ms/1(GbGDP_CCSMsgUpd_flg) -> Bus Creator/1  "GbGDP_CCSMsgUpd_flg"
  CEM_250ms/3(GeGDP_CEMToutBCP_enum) -> GeGDP_CEMToutBCP_enum/1
  CROUpdateClr_50ms/1(GbGDP_CROMsgUpd_flg) -> Bus Creator/6  "GbGDP_CROMsgUpd_flg"
  Bus Selector8/5 -> CSD_250ms/5(GcISP_3613ChrgrSer_numb)  "<GcISP_3613ChrgrSer_numb>"
  Bus Selector5/3 -> CRO_50ms/3(GcISP_2830ChrgrRdy_numb)  "<GcISP_2830ChrgrRdy_numb>"
  Bus Selector3/1 -> CHM_250ms/1(GbGDP_CHMMsgUpd_flg)  "<GbGDP_CHMMsgUpd_flg>"
  GDP_CTSUpdateClr_500ms/1 -> CTSUpdateClr_500ms/Trigger
  Bus Selector9/3 -> CEM_250ms/3(GeISP_3921ToutBRM_enum)  "<GeISP_3921ToutBRM_enum>"
  GDP_CHM_250ms/1 -> CHM_250ms/Trigger
  GcISP_2561ChrgrSer_numb/1 -> Bus Creator/11  "GcISP_2561ChrgrSer_numb"
  Bus Selector2/7 -> CTS_500ms/7(GcISP_2823SyncnMon_M)  "<GcISP_2823SyncnMon_M>"
  CST_10ms/14(GbGDP_ChrgrInFlt_flg) -> GbGDP_ChrgrInFlt_flg/1
  Bus Selector9/8 -> CEM_250ms/8(GeISP_3926ToutBST_enum)  "<GeISP_3926ToutBST_enum>"
  GcISP_2562ChrgrAr_numb/1 -> Bus Creator/12  "GcISP_2562ChrgrAr_numb"
  GDP_CCSUpdateClr_50ms/1 -> CCSUpdateClr_50ms/Trigger
  GcISP_2823SyncnDay_D/1 -> Bus Creator/16  "GcISP_2823SyncnDay_D"
  CTSUpdateClr_500ms/1(GbGDP_CTSMsgUpd_flg) -> Bus Creator/52  "GbGDP_CTSMsgUpd_flg"
  GDP_CSTUpdateClr_10ms/1 -> CSTUpdateClr_10ms/Trigger
  CEM_250ms/10(GbGDP_CEMToutFlt_flg) -> GbGDP_CEMToutFlt_flg/1
  Bus Selector7/10 -> CST_10ms/10(GeISP_3522OtherFlt_enum)  "<GeISP_3522OtherFlt_enum>"
  GDP_CROUpdateClr_50ms/1 -> CROUpdateClr_50ms/Trigger
  GeISP_3924ToutBCS_enum/1 -> Bus Creator/46  "GeISP_3924ToutBCS_enum"
  GDP_CST_10ms/1 -> CST_10ms/Trigger
  CCS_50ms/3(GcGDP_CCSCurOut_A) -> GcGDP_CCSCurOut_A/1
  GDP_CCS_50ms/1 -> CCS_50ms/Trigger
  GDP_CRMUpdateClr_250ms/1 -> CRMUpdateClr_250ms/Trigger
  CTS_500ms/7(GcGDP_CTSSyncnYr_Y) -> GcGDP_CTSSyncnYr_Y/1
  GcISP_2824ChrgrMaxVolt_V/1 -> Bus Creator/19  "GcISP_2824ChrgrMaxVolt_V"
  GcISP_2823SyncnMon_M/1 -> Bus Creator/17  "GcISP_2823SyncnMon_M"
  GeISP_3921ToutBRM_enum/1 -> Bus Creator/43  "GeISP_3921ToutBRM_enum"
  GeISP_3521ChrgrFlt_enum/1 -> Bus Creator/30  "GeISP_3521ChrgrFlt_enum"
  Bus Selector2/4 -> CTS_500ms/4(GcISP_2823SyncnMin_min)  "<GcISP_2823SyncnMin_min>"
  CEM_250ms/8(GeGDP_CEMToutBSD_enum) -> GeGDP_CEMToutBSD_enum/1
  CST_10ms/10(GeGDP_CSTChrgrOverTemp_enum) -> GeGDP_CSTChrgrOverTemp_enum/1
  GDP_CSDUpdateClr_250ms/1 -> CSDUpdateClr_250ms/Trigger
  CTS_500ms/3(GcGDP_CTSSyncnMin_min) -> GcGDP_CTSSyncnMin_min/1
  GDP_CHMUpdateClr_250ms/1 -> CHMUpdateClr_250ms/Trigger
  Bus Selector2/5 -> CTS_500ms/5(GcISP_2823SyncnHr_H)  "<GcISP_2823SyncnHr_H>"
  GeISP_3522ChrgrConntFlt_enum/1 -> Bus Creator/33  "GeISP_3522ChrgrConntFlt_enum"
  GDP_BusOff_10ms/1 -> BusOff_10ms/Trigger
  GeISP_3522CapDeliverFlt_enum/1 -> Bus Creator/32  "GeISP_3522CapDeliverFlt_enum"
  Bus Selector8/3 -> CSD_250ms/3(GcISP_3611SumChrgTi_min)  "<GcISP_3611SumChrgTi_min>"
  CTS_500ms/4(GcGDP_CTSSyncnHr_H) -> GcGDP_CTSSyncnHr_H/1
  GeISP_3523CurMismatch_enum/1 -> Bus Creator/38  "GeISP_3523CurMismatch_enum"
  Bus Selector2/2 -> CTS_500ms/2(GeDCC_DCConnSt_enum)  "<GeDCC_DCConnSt_enum>"
  GbISP_DCChrgCanNetStatus_flg/1 -> Bus Creator/54  "GbISP_DCChrgCanNetStatus_flg"
  Bus Selector10/2 -> BusOff_10ms/2(GbISP_DCChrgCanNetStatus_flg)  "<GbISP_DCChrgCanNetStatus_flg>"
  GeLDP_CC2St_enum/1 -> Bus Creator/55  "GeLDP_CC2St_enum"
  Bus Selector7/15 -> CST_10ms/15(GeLDP_CC2St_enum)  "<GeLDP_CC2St_enum>"
  Bus Selector9/11 -> CEM_250ms/11(GeLDP_CC2St_enum)  "<GeLDP_CC2St_enum>"
  GbLDP_DC12VSply_flg/1 -> CHM_250ms/4(GbLDP_DC12VSply_flg)

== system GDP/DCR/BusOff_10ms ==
  GbISP_DCCANBusOffFlt_flg : Inport
  GbISP_DCChrgCanNetStatus_flg : Inport  Port=2
  GDP_BusOff_10ms : TriggerPort  TriggerType=function-call  VariantControl=(inherit)
  BusOff_10ms_sys : Subsystem
  GbGDP_DCCANBusOffFlt_flg : Outport
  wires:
  BusOff_10ms_sys/1(GbGDP_DCCANBusOffFlt_flg) -> GbGDP_DCCANBusOffFlt_flg/1
  GbISP_DCCANBusOffFlt_flg/1 -> BusOff_10ms_sys/1(GbISP_DCCANBusOffFlt_flg)
  GbISP_DCChrgCanNetStatus_flg/1 -> BusOff_10ms_sys/2(GbISP_DCChrgCanNetStatus_flg)

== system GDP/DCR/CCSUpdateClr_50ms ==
  GDP_CCSUpdateClr_50ms : TriggerPort  TriggerType=function-call  VariantControl=(inherit)
  CCSUpdateClr_50ms_sys : Subsystem
  GbGDP_CCSMsgUpd_flg : Outport
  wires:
  CCSUpdateClr_50ms_sys/1(GbGDP_CCSMsgUpd_flg) -> GbGDP_CCSMsgUpd_flg/1

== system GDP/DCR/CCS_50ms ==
  GbGDP_CCSMsgUpd_flg : Inport
  GeDCC_DCConnSt_enum : Inport  Port=2
  GcISP_3081ChrgrVolt_V : Inport  Port=3
  GcISP_3082ChrgrCur_A : Inport  Port=4
  GcISP_3083ChrgTi_min : Inport  Port=5
  GeISP_3929ChrgrRdy_enum : Inport  Port=6
  GDP_CCS_50ms : TriggerPort  TriggerType=function-call  VariantControl=(inherit)
  CCS_50ms_sys : Subsystem
  GbGDP_CCSRecOnce_flg : Outport
  GcGDP_CCSVoltOut_V : Outport  Port=2
  GcGDP_CCSCurOut_A : Outport  Port=3
  GcGDP_CCSChrgrTime_min : Outport  Port=4
  GeGDP_CCSChrgrEN_enum : Outport  Port=5
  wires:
  GbGDP_CCSMsgUpd_flg/1 -> CCS_50ms_sys/1(GbGDP_CCSMsgUpd_flg)
  GeDCC_DCConnSt_enum/1 -> CCS_50ms_sys/2(GeDCC_DCConnSt_enum)
  GeISP_3929ChrgrRdy_enum/1 -> CCS_50ms_sys/6(GeISP_3929ChrgrRdy_enum)
  GcISP_3081ChrgrVolt_V/1 -> CCS_50ms_sys/3(GcISP_3081ChrgrVolt_V)
  GcISP_3083ChrgTi_min/1 -> CCS_50ms_sys/5(GcISP_3083ChrgTi_min)
  GcISP_3082ChrgrCur_A/1 -> CCS_50ms_sys/4(GcISP_3082ChrgrCur_A)
  CCS_50ms_sys/1(GbGDP_CCSRecOnce_flg) -> GbGDP_CCSRecOnce_flg/1
  CCS_50ms_sys/2(GcGDP_CCSVoltOut_V) -> GcGDP_CCSVoltOut_V/1
  CCS_50ms_sys/3(GcGDP_CCSCurOut_A) -> GcGDP_CCSCurOut_A/1
  CCS_50ms_sys/4(GcGDP_CCSChrgrTime_min) -> GcGDP_CCSChrgrTime_min/1
  CCS_50ms_sys/5(GeGDP_CCSChrgrEN_enum) -> GeGDP_CCSChrgrEN_enum/1

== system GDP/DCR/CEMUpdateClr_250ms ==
  GDP_CEMUpdateClr_250ms : TriggerPort  TriggerType=function-call  VariantControl=(inherit)
  CEMUpdateClr_250ms_sys : Subsystem
  GbGDP_CEMMsgUpd_flg : Outport
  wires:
  CEMUpdateClr_250ms_sys/1(GbGDP_CEMMsgUpd_flg) -> GbGDP_CEMMsgUpd_flg/1

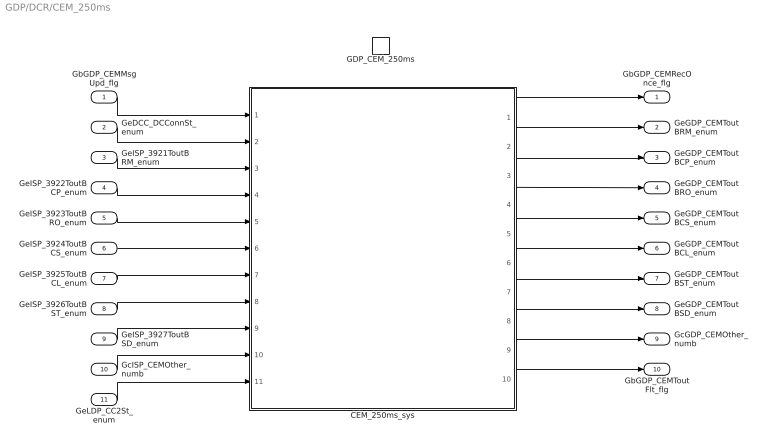
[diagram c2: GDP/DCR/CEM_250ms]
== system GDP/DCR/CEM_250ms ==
  GbGDP_CEMMsgUpd_flg : Inport
  GeDCC_DCConnSt_enum : Inport  Port=2
  GeISP_3921ToutBRM_enum : Inport  Port=3
  GeISP_3922ToutBCP_enum : Inport  Port=4
  GeISP_3923ToutBRO_enum : Inport  Port=5
  GeISP_3924ToutBCS_enum : Inport  Port=6
  GeISP_3925ToutBCL_enum : Inport  Port=7
  GeISP_3926ToutBST_enum : Inport  Port=8
  GeISP_3927ToutBSD_enum : Inport  Port=9
  GcISP_CEMOther_numb : Inport  Port=10
  GeLDP_CC2St_enum : Inport  Port=11
  GDP_CEM_250ms : TriggerPort  TriggerType=function-call  VariantControl=(inherit)
  CEM_250ms_sys : Subsystem
  GbGDP_CEMRecOnce_flg : Outport
  GeGDP_CEMToutBRM_enum : Outport  Port=2
  GeGDP_CEMToutBCP_enum : Outport  Port=3
  GeGDP_CEMToutBRO_enum : Outport  Port=4
  GeGDP_CEMToutBCS_enum : Outport  Port=5
  GeGDP_CEMToutBCL_enum : Outport  Port=6
  GeGDP_CEMToutBST_enum : Outport  Port=7
  GeGDP_CEMToutBSD_enum : Outport  Port=8
  GcGDP_CEMOther_numb : Outport  Port=9
  GbGDP_CEMToutFlt_flg : Outport  Port=10
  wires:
  GbGDP_CEMMsgUpd_flg/1 -> CEM_250ms_sys/1(GbGDP_CEMMsgUpd_flg)
  CEM_250ms_sys/1(GbGDP_CEMRecOnce_flg) -> GbGDP_CEMRecOnce_flg/1
  CEM_250ms_sys/2(GeGDP_CEMToutBRM_enum) -> GeGDP_CEMToutBRM_enum/1
  CEM_250ms_sys/3(GeGDP_CEMToutBCP_enum) -> GeGDP_CEMToutBCP_enum/1
  CEM_250ms_sys/4(GeGDP_CEMToutBRO_enum) -> GeGDP_CEMToutBRO_enum/1
  CEM_250ms_sys/5(GeGDP_CEMToutBCS_enum) -> GeGDP_CEMToutBCS_enum/1
  CEM_250ms_sys/6(GeGDP_CEMToutBCL_enum) -> GeGDP_CEMToutBCL_enum/1
  CEM_250ms_sys/7(GeGDP_CEMToutBST_enum) -> GeGDP_CEMToutBST_enum/1
  CEM_250ms_sys/8(GeGDP_CEMToutBSD_enum) -> GeGDP_CEMToutBSD_enum/1
  CEM_250ms_sys/9(GcGDP_CEMOther_numb) -> GcGDP_CEMOther_numb/1
  GeDCC_DCConnSt_enum/1 -> CEM_250ms_sys/2(GeDCC_DCConnSt_enum)
  GeISP_3924ToutBCS_enum/1 -> CEM_250ms_sys/6(GeISP_3924ToutBCS_enum)
  GeISP_3923ToutBRO_enum/1 -> CEM_250ms_sys/5(GeISP_3923ToutBRO_enum)
  GeISP_3925ToutBCL_enum/1 -> CEM_250ms_sys/7(GeISP_3925ToutBCL_enum)
  GeISP_3922ToutBCP_enum/1 -> CEM_250ms_sys/4(GeISP_3922ToutBCP_enum)
  GeISP_3921ToutBRM_enum/1 -> CEM_250ms_sys/3(GeISP_3921ToutBRM_enum)
  GeISP_3926ToutBST_enum/1 -> CEM_250ms_sys/8(GeISP_3926ToutBST_enum)
  GeISP_3927ToutBSD_enum/1 -> CEM_250ms_sys/9(GeISP_3927ToutBSD_enum)
  GcISP_CEMOther_numb/1 -> CEM_250ms_sys/10(GcISP_CEMOther_numb)
  CEM_250ms_sys/10(GbGDP_CEMToutFlt_flg) -> GbGDP_CEMToutFlt_flg/1
  GeLDP_CC2St_enum/1 -> CEM_250ms_sys/11(GeLDP_CC2St_enum)

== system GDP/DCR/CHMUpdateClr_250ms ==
  GDP_CHMUpdateClr_250ms : TriggerPort  TriggerType=function-call  VariantControl=(inherit)
  CHMUpdateClr_250ms_sys : Subsystem
  GbGDP_CHMMsgUpd_flg : Outport
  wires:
  CHMUpdateClr_250ms_sys/1(GbGDP_CHMMsgUpd_flg) -> GbGDP_CHMMsgUpd_flg/1

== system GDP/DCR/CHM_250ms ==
  GbGDP_CHMMsgUpd_flg : Inport
  GeDCC_DCConnSt_enum : Inport  Port=2
  GcISP_2600ChrgrVer_numb : Inport  Port=3
  GbLDP_DC12VSply_flg : Inport  Port=4
  GDP_CHM_250ms : TriggerPort  TriggerType=function-call  VariantControl=(inherit)
  CHM_250ms_sys : Subsystem
  GbGDP_CHMRecOnce_flg : Outport
  GcGDP_CHM2600ChrgrVer_numb : Outport  Port=2
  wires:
  GbGDP_CHMMsgUpd_flg/1 -> CHM_250ms_sys/1(GbGDP_CHMMsgUpd_flg)
  GeDCC_DCConnSt_enum/1 -> CHM_250ms_sys/2(GeDCC_DCConnSt_enum)
  GcISP_2600ChrgrVer_numb/1 -> CHM_250ms_sys/3(GcISP_2600ChrgrVer_numb)
  CHM_250ms_sys/1(GbGDP_CHMRecOnce_flg) -> GbGDP_CHMRecOnce_flg/1
  CHM_250ms_sys/2(GcGDP_CHM2600ChrgrVer_numb) -> GcGDP_CHM2600ChrgrVer_numb/1
  GbLDP_DC12VSply_flg/1 -> CHM_250ms_sys/4(GbLDP_DC12VSply_flg)

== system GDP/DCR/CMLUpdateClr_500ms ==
  GDP_CMLUpdateClr_500ms : TriggerPort  TriggerType=function-call  VariantControl=(inherit)
  CMLUpdateClr_500ms_sys : Subsystem
  GbGDP_CMLMsgUpd_flg : Outport
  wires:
  CMLUpdateClr_500ms_sys/1(GbGDP_CMLMsgUpd_flg) -> GbGDP_CMLMsgUpd_flg/1

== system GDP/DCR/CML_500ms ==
  GbGDP_CMLMsgUpd_flg : Inport
  GeDCC_DCConnSt_enum : Inport  Port=2
  GcISP_2824ChrgrMaxVolt_V : Inport  Port=3
  GcISP_2825ChrgrMinVolt_V : Inport  Port=4
  GcISP_2826ChrgrMaxCur_A : Inport  Port=5
  GcISP_2827ChrgrMinCur_A : Inport  Port=6
  GDP_CML_500ms : TriggerPort  TriggerType=function-call  VariantControl=(inherit)
  CML_500ms_sys : Subsystem
  GbGDP_CMLRecOnce_flg : Outport
  GcGDP_CMLChrgrMaxVolt_V : Outport  Port=2
  GcGDP_CMLChrgrMinVolt_V : Outport  Port=3
  GcGDP_CMLCurMaxOut_A : Outport  Port=4
  GcGDP_CMLCurMinOut_A : Outport  Port=5
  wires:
  GbGDP_CMLMsgUpd_flg/1 -> CML_500ms_sys/1(GbGDP_CMLMsgUpd_flg)
  GeDCC_DCConnSt_enum/1 -> CML_500ms_sys/2(GeDCC_DCConnSt_enum)
  GcISP_2824ChrgrMaxVolt_V/1 -> CML_500ms_sys/3(GcISP_2824ChrgrMaxVolt_V)
  GcISP_2825ChrgrMinVolt_V/1 -> CML_500ms_sys/4(GcISP_2825ChrgrMinVolt_V)
  GcISP_2826ChrgrMaxCur_A/1 -> CML_500ms_sys/5(GcISP_2826ChrgrMaxCur_A)
  GcISP_2827ChrgrMinCur_A/1 -> CML_500ms_sys/6(GcISP_2827ChrgrMinCur_A)
  CML_500ms_sys/1(GbGDP_CMLRecOnce_flg) -> GbGDP_CMLRecOnce_flg/1
  CML_500ms_sys/2(GcGDP_CMLChrgrMaxVolt_V) -> GcGDP_CMLChrgrMaxVolt_V/1
  CML_500ms_sys/3(GcGDP_CMLChrgrMinVolt_V) -> GcGDP_CMLChrgrMinVolt_V/1
  CML_500ms_sys/4(GcGDP_CMLCurMaxOut_A) -> GcGDP_CMLCurMaxOut_A/1
  CML_500ms_sys/5(GcGDP_CMLCurMinOut_A) -> GcGDP_CMLCurMinOut_A/1

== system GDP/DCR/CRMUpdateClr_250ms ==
  GDP_CRMUpdateClr_250ms : TriggerPort  TriggerType=function-call  VariantControl=(inherit)
  CRMUpdateClr_250ms_sys : Subsystem
  GbGDP_CRMMsgUpd_flg : Outport
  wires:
  CRMUpdateClr_250ms_sys/1(GbGDP_CRMMsgUpd_flg) -> GbGDP_CRMMsgUpd_flg/1

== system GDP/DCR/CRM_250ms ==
  GbGDP_CRMMsgUpd_flg : Inport
  GeDCC_DCConnSt_enum : Inport  Port=2
  GcISP_2560ChrgrAck_numb : Inport  Port=3
  GcISP_2561ChrgrSer_numb : Inport  Port=4
  GcISP_2562ChrgrAr_numb : Inport  Port=5
  GDP_CRM_250ms : TriggerPort  TriggerType=function-call  VariantControl=(inherit)
  CRM_250ms_sys : Subsystem
  GbGDP_CRMRecOnce_flg : Outport
  GcGDP_CRMChrgrAck_numb : Outport  Port=2
  GcGDP_CRMChrgrAr_numb : Outport  Port=3
  GcGDP_CRMChrgrSer_numb : Outport  Port=4
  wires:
  GbGDP_CRMMsgUpd_flg/1 -> CRM_250ms_sys/1(GbGDP_CRMMsgUpd_flg)
  GeDCC_DCConnSt_enum/1 -> CRM_250ms_sys/2(GeDCC_DCConnSt_enum)
  GcISP_2560ChrgrAck_numb/1 -> CRM_250ms_sys/3(GcISP_2560ChrgrAck_numb)
  CRM_250ms_sys/1(GbGDP_CRMRecOnce_flg) -> GbGDP_CRMRecOnce_flg/1
  CRM_250ms_sys/2(GcGDP_CRMChrgrAck_numb) -> GcGDP_CRMChrgrAck_numb/1
  GcISP_2561ChrgrSer_numb/1 -> CRM_250ms_sys/4(GcISP_2561ChrgrSer_numb)
  GcISP_2562ChrgrAr_numb/1 -> CRM_250ms_sys/5(GcISP_2562ChrgrAr_numb)
  CRM_250ms_sys/3(GcGDP_CRMChrgrAr_numb) -> GcGDP_CRMChrgrAr_numb/1
  CRM_250ms_sys/4(GcGDP_CRMChrgrSer_numb) -> GcGDP_CRMChrgrSer_numb/1

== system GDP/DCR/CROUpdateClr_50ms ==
  GDP_CROUpdateClr_50ms : TriggerPort  TriggerType=function-call  VariantControl=(inherit)
  CROUpdateClr_50ms_sys : Subsystem
  GbGDP_CROMsgUpd_flg : Outport
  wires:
  CROUpdateClr_50ms_sys/1(GbGDP_CROMsgUpd_flg) -> GbGDP_CROMsgUpd_flg/1

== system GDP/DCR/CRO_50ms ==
  GbGDP_CROMsgUpd_flg : Inport
  GeDCC_DCConnSt_enum : Inport  Port=2
  GcISP_2830ChrgrRdy_numb : Inport  Port=3
  GDP_CRO_50ms : TriggerPort  TriggerType=function-call  VariantControl=(inherit)
  CRO_50ms_sys : Subsystem
  GbGDP_CRORecOnce_flg : Outport
  GcGDP_CROChrgrRdy_numb : Outport  Port=2
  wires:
  GbGDP_CROMsgUpd_flg/1 -> CRO_50ms_sys/1(GbGDP_CROMsgUpd_flg)
  GeDCC_DCConnSt_enum/1 -> CRO_50ms_sys/2(GeDCC_DCConnSt_enum)
  GcISP_2830ChrgrRdy_numb/1 -> CRO_50ms_sys/3(GcISP_2830ChrgrRdy_numb)
  CRO_50ms_sys/1(GbGDP_CRORecOnce_flg) -> GbGDP_CRORecOnce_flg/1
  CRO_50ms_sys/2(GcGDP_CROChrgrRdy_numb) -> GcGDP_CROChrgrRdy_numb/1

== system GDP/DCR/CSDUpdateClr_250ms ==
  GDP_CSDUpdateClr_250ms : TriggerPort  TriggerType=function-call  VariantControl=(inherit)
  CSDUpdateClr_250ms_sys : Subsystem
  GbGDP_CSDMsgUpd_flg : Outport
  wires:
  CSDUpdateClr_250ms_sys/1(GbGDP_CSDMsgUpd_flg) -> GbGDP_CSDMsgUpd_flg/1

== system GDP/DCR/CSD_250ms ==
  GbGDP_CSDMsgUpd_flg : Inport
  GeDCC_DCConnSt_enum : Inport  Port=2
  GcISP_3611SumChrgTi_min : Inport  Port=3
  GcISP_3612SumEgy_kWh : Inport  Port=4
  GcISP_3613ChrgrSer_numb : Inport  Port=5
  GDP_CSD_250ms : TriggerPort  TriggerType=function-call  VariantControl=(inherit)
  CSD_250ms_sys : Subsystem
  GbGDP_CSDRecOnce_flg : Outport
  GcGDP_CSDSumChrgTi_min : Outport  Port=2
  GcGDP_CSDSumEgy_kWh : Outport  Port=3
  GcGDP_CSDChrgrSer_numb : Outport  Port=4
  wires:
  GbGDP_CSDMsgUpd_flg/1 -> CSD_250ms_sys/1(GbGDP_CSDMsgUpd_flg)
  GeDCC_DCConnSt_enum/1 -> CSD_250ms_sys/2(GeDCC_DCConnSt_enum)
  GcISP_3611SumChrgTi_min/1 -> CSD_250ms_sys/3(GcISP_3611SumChrgTi_min)
  GcISP_3612SumEgy_kWh/1 -> CSD_250ms_sys/4(GcISP_3612SumEgy_kWh)
  GcISP_3613ChrgrSer_numb/1 -> CSD_250ms_sys/5(GcISP_3613ChrgrSer_numb)
  CSD_250ms_sys/1(GbGDP_CSDRecOnce_flg) -> GbGDP_CSDRecOnce_flg/1
  CSD_250ms_sys/2(GcGDP_CSDSumChrgTi_min) -> GcGDP_CSDSumChrgTi_min/1
  CSD_250ms_sys/3(GcGDP_CSDSumEgy_kWh) -> GcGDP_CSDSumEgy_kWh/1
  CSD_250ms_sys/4(GcGDP_CSDChrgrSer_numb) -> GcGDP_CSDChrgrSer_numb/1

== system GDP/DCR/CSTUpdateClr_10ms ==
  GDP_CSTUpdateClr_10ms : TriggerPort  TriggerType=function-call  VariantControl=(inherit)
  CSTUpdateClr_10ms_sys : Subsystem
  GbGDP_CSTMsgUpd_flg : Outport
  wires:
  CSTUpdateClr_10ms_sys/1(GbGDP_CSTMsgUpd_flg) -> GbGDP_CSTMsgUpd_flg/1

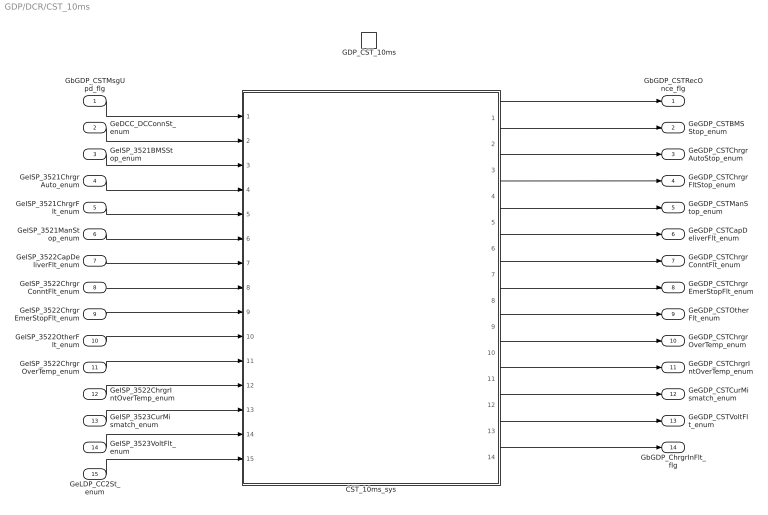
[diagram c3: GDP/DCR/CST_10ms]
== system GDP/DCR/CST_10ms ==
  GbGDP_CSTMsgUpd_flg : Inport
  GeDCC_DCConnSt_enum : Inport  Port=2
  GeISP_3521BMSStop_enum : Inport  Port=3
  GeISP_3521ChrgrAuto_enum : Inport  Port=4
  GeISP_3521ChrgrFlt_enum : Inport  Port=5
  GeISP_3521ManStop_enum : Inport  Port=6
  GeISP_3522CapDeliverFlt_enum : Inport  Port=7
  GeISP_3522ChrgrConntFlt_enum : Inport  Port=8
  GeISP_3522ChrgrEmerStopFlt_enum : Inport  Port=9
  GeISP_3522OtherFlt_enum : Inport  Port=10
  GeISP_3522ChrgrOverTemp_enum : Inport  Port=11
  GeISP_3522ChrgrIntOverTemp_enum : Inport  Port=12
  GeISP_3523CurMismatch_enum : Inport  Port=13
  GeISP_3523VoltFlt_enum : Inport  Port=14
  GeLDP_CC2St_enum : Inport  Port=15
  GDP_CST_10ms : TriggerPort  TriggerType=function-call  VariantControl=(inherit)
  CST_10ms_sys : Subsystem
  GbGDP_CSTRecOnce_flg : Outport
  GeGDP_CSTBMSStop_enum : Outport  Port=2
  GeGDP_CSTChrgrAutoStop_enum : Outport  Port=3
  GeGDP_CSTChrgrFltStop_enum : Outport  Port=4
  GeGDP_CSTManStop_enum : Outport  Port=5
  GeGDP_CSTCapDeliverFlt_enum : Outport  Port=6
  GeGDP_CSTChrgrConntFlt_enum : Outport  Port=7
  GeGDP_CSTChrgrEmerStopFlt_enum : Outport  Port=8
  GeGDP_CSTOtherFlt_enum : Outport  Port=9
  GeGDP_CSTChrgrOverTemp_enum : Outport  Port=10
  GeGDP_CSTChrgrIntOverTemp_enum : Outport  Port=11
  GeGDP_CSTCurMismatch_enum : Outport  Port=12
  GeGDP_CSTVoltFlt_enum : Outport  Port=13
  GbGDP_ChrgrInFlt_flg : Outport  Port=14
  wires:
  GbGDP_CSTMsgUpd_flg/1 -> CST_10ms_sys/1(GbGDP_CSTMsgUpd_flg)
  GeDCC_DCConnSt_enum/1 -> CST_10ms_sys/2(GeDCC_DCConnSt_enum)
  GeISP_3521BMSStop_enum/1 -> CST_10ms_sys/3(GeISP_3521BMSStop_enum)
  GeISP_3521ChrgrAuto_enum/1 -> CST_10ms_sys/4(GeISP_3521ChrgrAuto_enum)
  GeISP_3521ChrgrFlt_enum/1 -> CST_10ms_sys/5(GeISP_3521ChrgrFlt_enum)
  GeISP_3521ManStop_enum/1 -> CST_10ms_sys/6(GeISP_3521ManStop_enum)
  GeISP_3522CapDeliverFlt_enum/1 -> CST_10ms_sys/7(GeISP_3522CapDeliverFlt_enum)
  GeISP_3522ChrgrConntFlt_enum/1 -> CST_10ms_sys/8(GeISP_3522ChrgrConntFlt_enum)
  GeISP_3522ChrgrEmerStopFlt_enum/1 -> CST_10ms_sys/9(GeISP_3522ChrgrEmerStopFlt_enum)
  GeISP_3522OtherFlt_enum/1 -> CST_10ms_sys/10(GeISP_3522OtherFlt_enum)
  GeISP_3522ChrgrOverTemp_enum/1 -> CST_10ms_sys/11(GeISP_3522ChrgrOverTemp_enum)
  GeISP_3522ChrgrIntOverTemp_enum/1 -> CST_10ms_sys/12(GeISP_3522ChrgrIntOverTemp_enum)
  GeISP_3523CurMismatch_enum/1 -> CST_10ms_sys/13(GeISP_3523CurMismatch_enum)
  GeISP_3523VoltFlt_enum/1 -> CST_10ms_sys/14(GeISP_3523VoltFlt_enum)
  CST_10ms_sys/1(GbGDP_CSTRecOnce_flg) -> GbGDP_CSTRecOnce_flg/1
  CST_10ms_sys/2(GeGDP_CSTBMSStop_enum) -> GeGDP_CSTBMSStop_enum/1
  CST_10ms_sys/3(GeGDP_CSTChrgrAutoStop_enum) -> GeGDP_CSTChrgrAutoStop_enum/1
  CST_10ms_sys/4(GeGDP_CSTChrgrFltStop_enum) -> GeGDP_CSTChrgrFltStop_enum/1
  CST_10ms_sys/5(GeGDP_CSTManStop_enum) -> GeGDP_CSTManStop_enum/1
  CST_10ms_sys/6(GeGDP_CSTCapDeliverFlt_enum) -> GeGDP_CSTCapDeliverFlt_enum/1
  CST_10ms_sys/7(GeGDP_CSTChrgrConntFlt_enum) -> GeGDP_CSTChrgrConntFlt_enum/1
  CST_10ms_sys/8(GeGDP_CSTChrgrEmerStopFlt_enum) -> GeGDP_CSTChrgrEmerStopFlt_enum/1
  CST_10ms_sys/9(GeGDP_CSTOtherFlt_enum) -> GeGDP_CSTOtherFlt_enum/1
  CST_10ms_sys/12(GeGDP_CSTCurMismatch_enum) -> GeGDP_CSTCurMismatch_enum/1
  CST_10ms_sys/13(GeGDP_CSTVoltFlt_enum) -> GeGDP_CSTVoltFlt_enum/1
  CST_10ms_sys/11(GeGDP_CSTChrgrIntOverTemp_enum) -> GeGDP_CSTChrgrIntOverTemp_enum/1
  CST_10ms_sys/10(GeGDP_CSTChrgrOverTemp_enum) -> GeGDP_CSTChrgrOverTemp_enum/1
  CST_10ms_sys/14(GbGDP_ChrgrInFlt_flg) -> GbGDP_ChrgrInFlt_flg/1
  GeLDP_CC2St_enum/1 -> CST_10ms_sys/15(GeLDP_CC2St_enum)

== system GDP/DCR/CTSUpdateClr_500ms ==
  GDP_CTSUpdateClr_500ms : TriggerPort  TriggerType=function-call  VariantControl=(inherit)
  CTSUpdateClr_500ms_sys : Subsystem
  GbGDP_CTSMsgUpd_flg : Outport
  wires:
  CTSUpdateClr_500ms_sys/1(GbGDP_CTSMsgUpd_flg) -> GbGDP_CTSMsgUpd_flg/1
